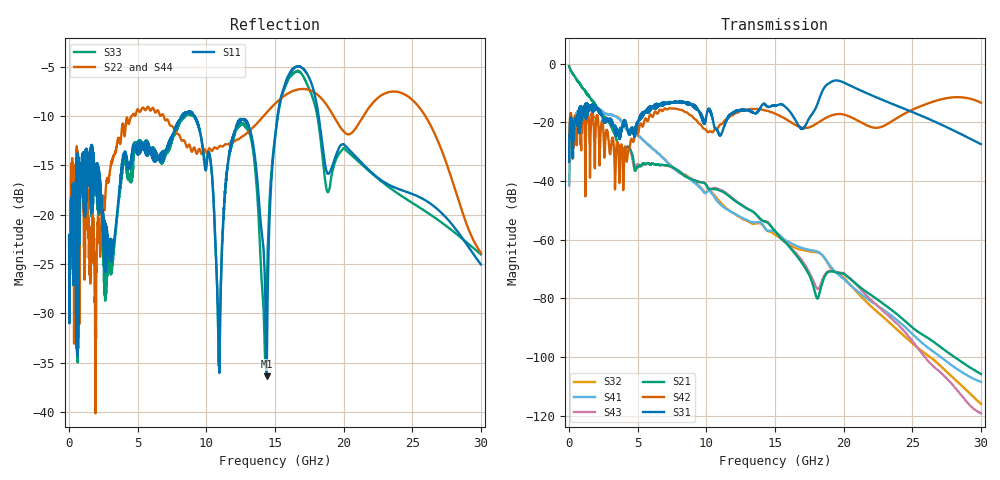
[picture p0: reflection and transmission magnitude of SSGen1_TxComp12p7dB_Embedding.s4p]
# Hz S RI R 50
! S-Parameters data
! Freq  reS11  imS11  reS12  imS12  reS13  imS13  reS14  imS14
!  reS21  imS21  reS22  imS22  reS23  imS23  reS24  imS24
!  reS31  imS31  reS32  imS32  reS33  imS33  reS34  imS34
!  reS41  imS41  reS42  imS42  reS43  imS43  reS44  imS44
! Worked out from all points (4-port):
!   1500 points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, 20 MHz to 30 GHz, reference 50 ohm
!   strongest paths, dB at 20 MHz, 7.52 GHz, 15.02 GHz, 22.52 GHz, 30 GHz:
!     S31: -33.5, -13.2, -14.3, -11.8, -27.4
!     S42: -29.2, -15.3, -17.1, -21.8, -13.3
!     S21: -0.9, -35.2, -57.1, -80.6, -105.8
!     S43: -0.9, -35.4, -57.2, -82.8, -119.2
!     S41: -41.5, -35.3, -57.4, -82.7, -108.5
!     S32: -41.5, -35.3, -58.4, -84.9, -115.9
!   lowest |S11| = -36.4 dB at 14.4 GHz (marker M1), VSWR 1.03, Z = 51.3 + j0.842 ohm
!   |S11| at or under -10 dB: start of sweep to 8.199 GHz; 9.161 GHz to 15.19 GHz (6.033 GHz wide, 49.5 % of centre); 18.19 GHz to end of sweep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
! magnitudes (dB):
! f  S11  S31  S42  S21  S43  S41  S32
! 20 MHz  -22.1  -33.5  -29.2  -0.9  -0.9  -41.5  -41.5
! 2.08 GHz  -14.8  -15.2  -17.7  -15.0  -15.0  -15.6  -15.7
! 10.94 GHz  -34.5  -24.0  -21.2  -43.2  -42.8  -47.5  -46.8
! 12.84 GHz  -10.5  -16.0  -15.7  -49.0  -48.9  -53.0  -53.4
! 14.4 GHz  -36.4  -14.4  -16.0  -54.0  -53.8  -56.7  -56.9
! 16.6 GHz  -5.0  -20.1  -21.2  -65.6  -65.0  -62.2  -63.0
! 30 GHz  -25.0  -27.4  -13.3  -105.8  -119.2  -108.5  -115.9
